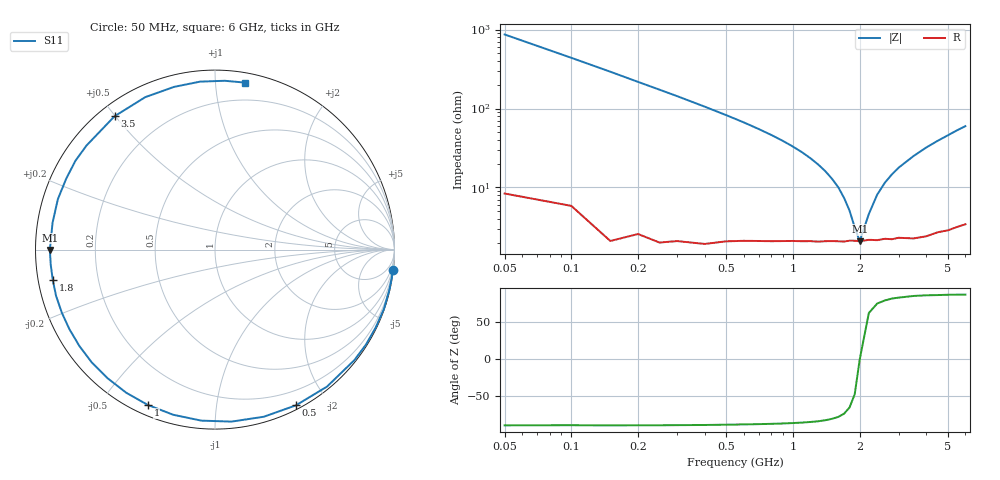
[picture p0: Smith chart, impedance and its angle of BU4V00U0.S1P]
! Infineon Technologies  Discrete & RF Semiconductors
! BB 833
! Si Tuning Diode in SOD323
! VR = 4 V
! S-Parameters:  June  1999
# GHz  S  MA  R  50
!  f  S11
! GHz  MAG  ANG
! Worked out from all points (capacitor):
!   34 points, 50 MHz to 6 GHz, reference 50 ohm
!   read as one part to ground: C = 3.62 pF near 50 MHz
!   lowest |Z| = 2.08 ohm at 2 GHz (marker M1)
!   series resonance near 2.002 GHz, so ESL is about 1.7 nH
!   S11 on the Smith chart (normalised r, x): 50 MHz: 0, -17; 500 MHz: 0.04, -1.65; 1 GHz: 0.04, -0.66; 1.8 GHz: 0.04, -0.09; 3.5 GHz: 0.05, +0.50; 6 GHz: 0.07, +1.19
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0.05  0.9989 -6.6
0.15  0.9976 -19.4
0.25  0.9939 -32.2
0.3  0.991 -38.4
0.4  0.986 -50.7
0.5  0.9779 -62.5
0.6  0.9701 -73.7
0.7  0.9628 -84.5
0.8  0.9559 -94.6
0.9  0.9492 -104.2
1  0.9431 -113.3
1.1  0.9384 -121.8
1.2  0.9337 -129.9
1.3  0.931 -137.5
1.5  0.9244 -151.4
1.6  0.923 -157.6
1.8  0.9194 -169.4
2  0.9201 -179.9
2.2  0.9173 170.7
2.4  0.9195 162.2
2.8  0.9217 147.5
3  0.9213 141.0
3.5  0.9301 127.0
4  0.9341 114.6
4.5  0.9348 104.1
5  0.9395 95.1
5.5  0.9422 86.7
6  0.9453 79.8
